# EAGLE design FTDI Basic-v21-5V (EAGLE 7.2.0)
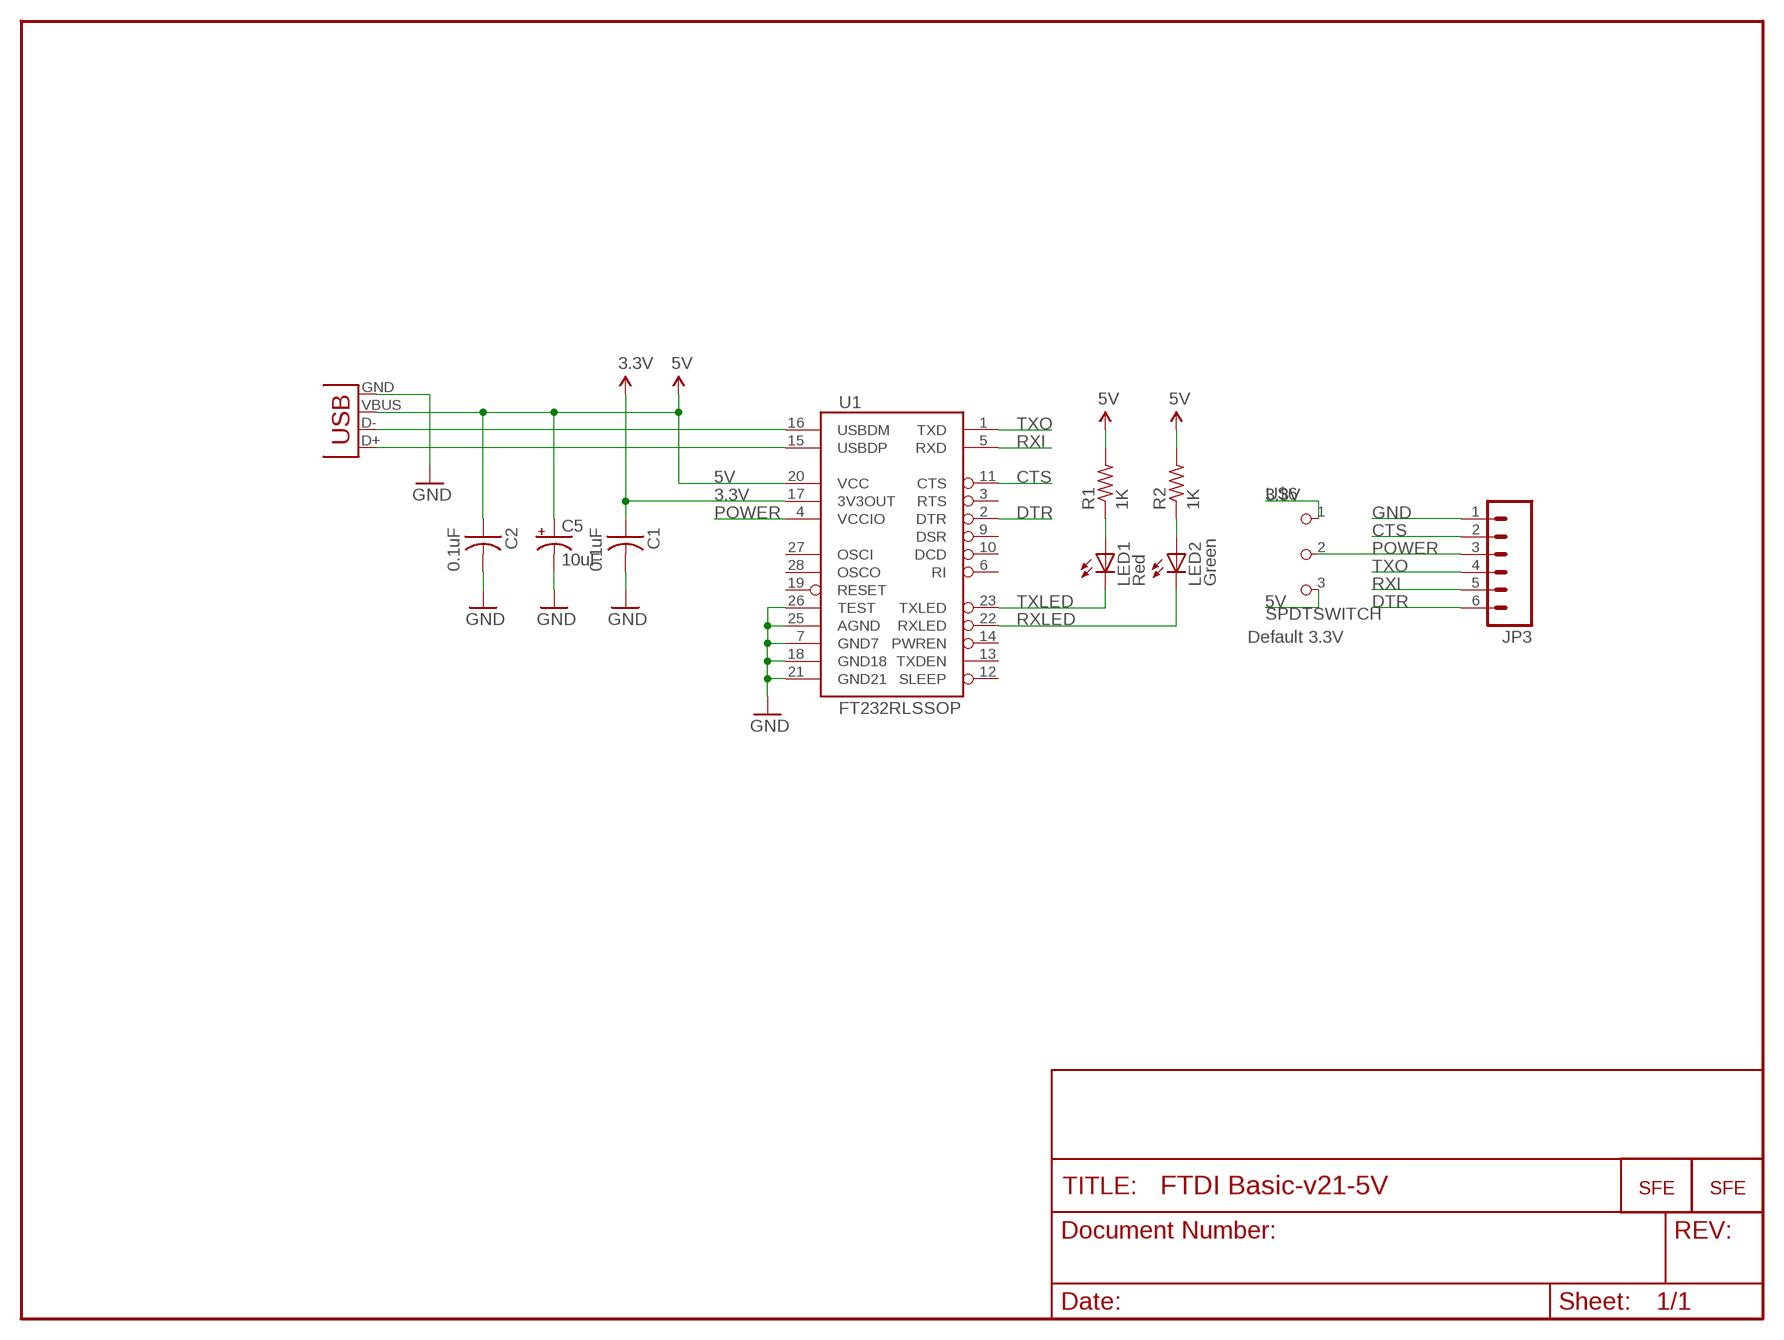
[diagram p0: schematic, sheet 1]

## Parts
C1  0.1uF  CAP-US1206FAB  [C1206FAB]
C2  0.1uF  CAP-US1206FAB  [C1206FAB]
C5  10uF  CAP_POL1206  [EIA3216]
JP2  LOGO-SFESK  [SFE-LOGO-FLAME]
JP3  M06SMD  [1X06-SMD]
LED1  Red  LEDSMT1206  [1206]
LED2  Green  LEDSMT1206  [1206]
R1  1K  RES-US1206FAB  [R1206FAB]
R2  1K  RES-US1206FAB  [R1206FAB]
U1  FT232RLSSOP  [SSOP28DB]
U$2  LOGO-SFENW2  [SFE-NEW-WEB]
U$5  USB_MINIB  [USB_MINIB]
U$6  SPDTSWITCH  [SPDTSWITCH]

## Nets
3.3V [power]: C1.1 U1.17(3V3OUT) U$6.1
5V: C2.1 C5.A(+) R1.2 R2.2 U1.20(VCC) U$5.VBUS U$6.3
CTS: JP3.2 U1.11(CTS)
DTR: JP3.6 U1.2(DTR)
GND [power]: C1.2 C2.2 C5.C(-) JP3.1 U1.7(GND7) U1.18(GND18) U1.21(GND21) U1.25(AGND) U1.26(TEST) U$5.GND
N$1: LED1.A R1.1
N$2: LED2.A R2.1
POWER: JP3.3 U1.4(VCCIO) U$6.2
RXI: JP3.5 U1.5(RXD)
RXLED: LED2.C U1.22(RXLED)
TXLED: LED1.C U1.23(TXLED)
TXO: JP3.4 U1.1(TXD)
USB_D+: U1.15(USBDP) U$5.D+
USB_D-: U1.16(USBDM) U$5.D-
Unconnected: U1.3(RTS) U1.6(RI) U1.9(DSR) U1.10(DCD) U1.12(SLEEP) U1.13(TXDEN) U1.14(PWREN) U1.19(RESET) U1.27(OSCI) U1.28(OSCO)

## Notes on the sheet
- Default 3.3V

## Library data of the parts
C1 C2 = fab:CAP-US
C5 = SparkFun:CAP_POL: Capacitor Polarized
JP2 U$2 = SparkFun:LOGO-SFE: Spark Fun Electronics PCB Logo
JP3 = 01_SparkFun:M06: Header 6 Standard 6-pin 0.1" header. Use with straight break away headers (SKU : PRT-00116), right angle break away headers (PRT-00553), swiss pins (PRT-00743), machine pins (PRT-00117), and female headers (PRT-00115). Molex polarized connector foot print use with SKU : PRT-08094 with associated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
LED1 LED2 = adafruit:LED: LED
R1 R2 = fab:RES-US: Resistor (US Symbol)
U1 = SparkFun:FT232RL: USB UART FT232RL 4th Generation USB UART (USB <-> Serial) Controller. Spark Fun Electronics SKU : COM-00650
U$5 = 01_fab:USB_MINIB
U$6 = fab:SPDTSWITCH

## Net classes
0 default: width 0.203 mm
1 power: width 0.254 mm

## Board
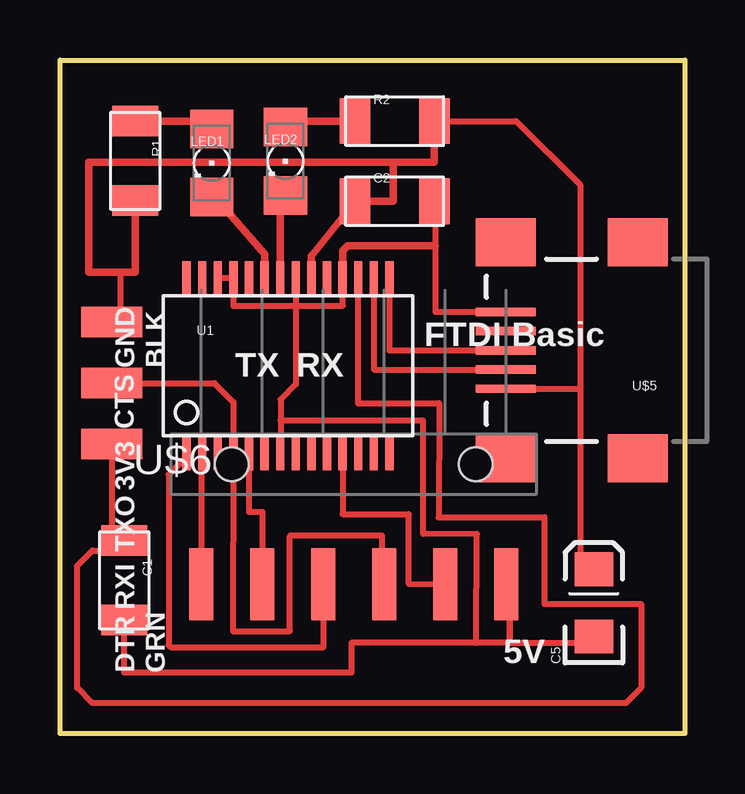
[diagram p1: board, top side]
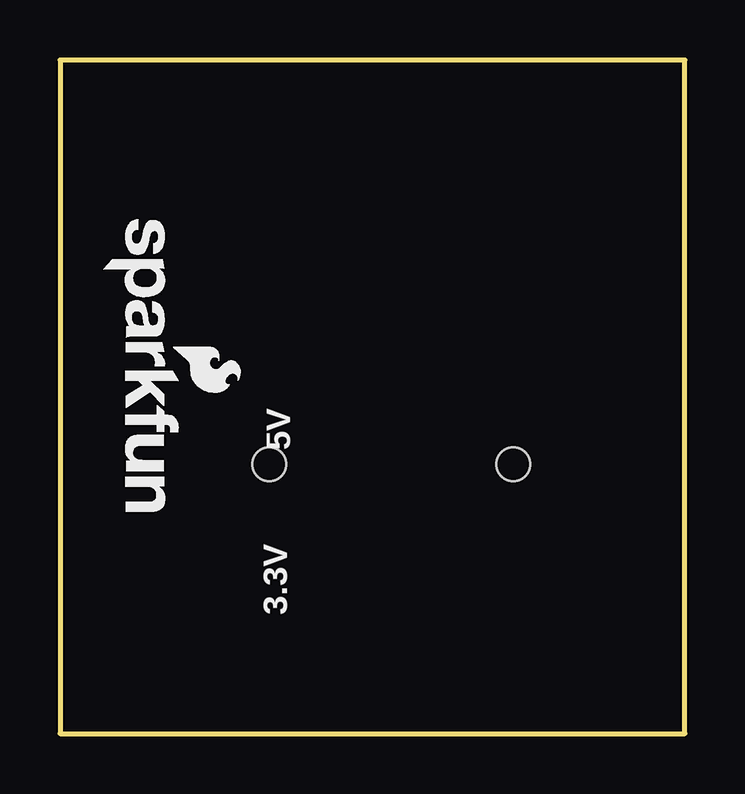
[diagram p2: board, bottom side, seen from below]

Size 26.04 x 28.07 mm. Coordinates in mm from the lower left corner, seen from the top.
Outline: 26.04,28.07 26.04,0 0,0 0,28.07 26.04,28.07
Copper layers (1*16): Top 0.035mm / dielectric 1.5mm / Bottom 0.035mm
Design rules "SparkFun *": minimum track width 8mil, minimum drill 20mil, track to track 10mil, track to pad 10mil, pad to pad 10mil, via to via 8mil, smd to smd 8mil, copper to edge 8mil, drill to drill 8mil, minimum pad ring 12mil, minimum via ring 10mil, stop-mask expansion 4mil, vias tented up to drill 20mil, thermal gap 10mil

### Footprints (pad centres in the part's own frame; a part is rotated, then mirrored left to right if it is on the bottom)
C1206FAB = smd 1.27 x 1.905: 1 -1.651,0; 2 1.651,0
EIA3216 = smd 1.4 x 1.6: A 1.4,0; C -1.4,0
1X06-SMD = smd 1 x 3: 1 -6.35,5; 2 -3.81,5; 3 -1.27,5; 4 1.27,5; 5 3.81,5; 6 6.35,5 | hole 1.4: -5.08,0; 5.08,0
1206 = smd 1.6 x 1.803: A -1.422,0; C 1.422,0
R1206FAB = smd 1.27 x 1.905: 1 -1.651,0; 2 1.651,0
SSOP28DB = smd 0.348 x 1.397: 1 -4.225,-3.656; 2 -3.575,-3.656; 3 -2.925,-3.656; 4 -2.275,-3.656; 5 -1.625,-3.656; 6 -0.975,-3.656; 7 -0.325,-3.656; 8 0.325,-3.656; 9 0.975,-3.656; 10 1.625,-3.656; 11 2.275,-3.656; 12 2.925,-3.656; 13 3.575,-3.656; 14 4.225,-3.656; 15 4.225,3.656; 16 3.575,3.656; 17 2.925,3.656; 18 2.275,3.656; 19 1.625,3.656; 20 0.975,3.656; 21 0.325,3.656; 22 -0.325,3.656; 23 -0.975,3.656; 24 -1.625,3.656; 25 -2.275,3.656; 26 -2.925,3.656; 27 -3.575,3.656; 28 -4.225,3.656
USB_MINIB = smd 2.5 x 0.35: D+ 3.77,0; D- 3.77,0.8; GND 3.77,-1.6; ID 3.77,-0.8; VBUS 3.77,1.6 | smd 2.5 x 2: GND@1 -1.73,-4.5; GND@2 -1.73,4.5; GND@3 3.77,4.5; GND@4 3.77,-4.5
SPDTSWITCH = smd 2.54 x 1.27: 1 0.38,2.54; 2 0.38,0; 3 0.38,-2.54

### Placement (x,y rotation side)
C1  2.67,6.39 270 top
C2  13.94,22.19 0 top
C5  22.24,5.45 90 top
JP2  21.31,16.09 270 bottom
JP3  12.24,11.22 180 top
LED1  6.32,23.77 270 top
LED2  9.39,23.85 270 top
R1  3.13,23.87 270 top
R2  13.94,25.52 0 top
U1  9.5,15.33 0 top
U$2  24.23,21.42 270 bottom
U$5  22.33,15.97 180 top
U$6  2.54,14.61 180 top

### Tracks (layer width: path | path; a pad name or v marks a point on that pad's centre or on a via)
3.3V
  Top 0.254: U1.17 12.41,13.76 15.79,13.77 15.78,9.01 20.19,9.02 20.19,5.4 24.21,5.4 24.21,1.91 23.57,1.27 1.35,1.27 0.71,1.91 0.71,6.99 1.35,7.62 2.26,7.62 C1.1 | 3.02,8.38 C1.1 | U$6.1 2.16,8.55 C1.1
5V
  Top 0.254: R2.2 19.01,25.52 21.67,22.86 21.67,14.37 | U$5.VBUS 21.67,14.37 | 21.67,14.37 21.67,6.99 22.24,6.99 C5.A | U$6.3 2.54,17.14 2.54,19.22
  Top 0.305: R1.2 3.13,19.22 2.54,19.22 1.19,19.22 1.19,23.81 13.89,23.81 | U1.20 10.47,19.89 C2.1 13.89,22.19 13.89,23.81 | 13.89,23.81 15.6,23.81 R2.2
CTS
  Top 0.254: U1.11 11.78,9.14 14.52,9.14 14.53,9.13 14.53,6.24 JP3.2
DTR
  Top 0.254: U1.2 5.89,11.67 JP3.6
GND
  Top 0.254: C2.2 15.64,21.55 15.64,20.32 15.64,17.57 16.98,17.57 U$5.GND | U1.26 U1.25 7.22,17.82 9.83,17.82 9.83,17.83 | 9.2,13.04 9.2,13.92 9.82,14.55 U1.21 9.83,17.83 | 9.2,13.04 9.2,11.69 U1.7 | 9.83,17.83 11.79,17.83 11.79,18.98 U1.18 | 18.74,3.77 18.74,5.13 JP3.1 18.73,6.22 18.73,3.81 | 18.74,3.77 17.35,3.77 | 17.35,3.77 17.37,8.32 15.14,8.32 15.13,13.04 9.2,13.04 | 22.3,3.65 22.3,3.81 21.67,3.81 21.67,4.05 C5.C 22.24,3.77 18.74,3.77 | 17.35,3.77 12.14,3.77 12.14,2.54 2.67,2.54 C1.2
  Top 0.305: U1.18 11.78,20.11 11.99,20.32 15.64,20.32
N$1
  Top 0.305: 6.33,25.52 R1.1
  Top 0.406: 6.33,25.52 LED1.A
N$2
  Top 0.305: R2.1 9.8,25.52 LED2.A
POWER
  Top 0.254: U1.4 | U1.4 7.21,4.27 9.58,4.27 9.58,8.23 9.6,8.26 13.41,8.26 13.41,6.32 JP3.3 | U1.4 | U$6.2 6.43,14.61 7.22,13.81 U1.4
RXI
  Top 0.254: U1.5 7.88,9.24 8.43,9.24 JP3.5
RXLED
  Top 0.305: LED2.C 9.18,22.21 U1.22
TXLED
  Top 0.305: LED1.C 6.46,22.35 8.53,19.97 U1.23
TXO
  Top 0.254: JP3.4 10.98,3.61 4.61,3.61 4.52,3.69 4.52,10.79 5.28,11.54 U1.1
USB_D+
  Top 0.254: U1.15 13.72,15.97 U$5.D+
USB_D-
  Top 0.254: U1.16 13.07,15.17 U$5.D-

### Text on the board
tPlace: FTDI Basic | GND | BLK | TX | RX | CTS | 3V3 | TXO | RXI | DTR | GRN | 5V
bPlace: 5V | 3.3V
tValues: Close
